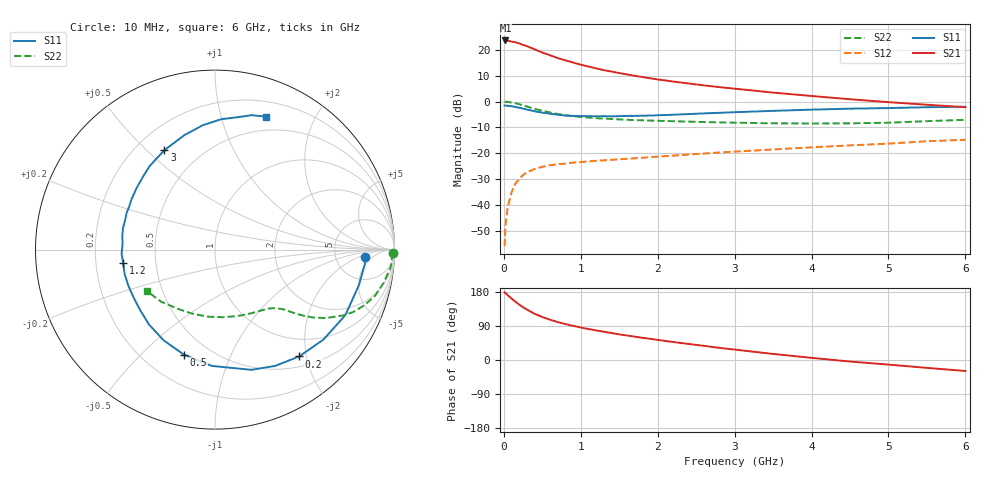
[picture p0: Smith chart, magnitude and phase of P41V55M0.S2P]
! SIEMENS Small Signal Semiconductors
! BFP182
! Si NPN RF Bipolar Junction Transistor in SOT143
! VCE = 1.5 V  IC = 5 mA
! Common Emitter S-Parameters:  March  1996
# GHz  S  MA  R  50
!  f  S11  S21  S12  S22
! GHz  MAG  ANG  MAG  ANG  MAG  ANG  MAG  ANG
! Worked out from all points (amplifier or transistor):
!   36 points, 10 MHz to 6 GHz, reference 50 ohm
!   highest |S21| = 23.6 dB at 20 MHz (marker M1)
!   |S21| within 3 dB of that: start of sweep to 364.8 MHz
!   unconditionally stable (mu >= 1): 1.537 GHz to 5.616 GHz
!   at 250 MHz: K = 0.22, MSG = 25.1 dB, |S12| = -28.4 dB
!   at 1.4 GHz: K = 0.95, MSG = 17.0 dB, |S12| = -22.5 dB
!   at 6 GHz: K = 0.96, MSG = 6.3 dB, |S12| = -14.8 dB
!   S11 on the Smith chart (normalised r, x): 10 MHz: 10, -3; 200 MHz: 0.67, -1.87; 500 MHz: 0.37, -0.68; 1.2 GHz: 0.32, -0.07; 3 GHz: 0.31, +0.57; 6 GHz: 0.35, +1.40
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0.01  0.8356 -2.8  14.93 178.4  0.0016 89.8  0.9898 -1.1
0.02  0.8386 -5.6  15.16 176.8  0.0039 89.9  0.9877 -2.2
0.05  0.8258 -13.9  15.03 170.9  0.0091 87.2  0.9838 -5.7
0.1  0.8129 -26.7  14.42 162.2  0.0176 74.6  0.9581 -11.1
0.15  0.785 -39.7  13.99 153.7  0.0257 68.8  0.9272 -16.2
0.2  0.7578 -51.8  13.29 146.1  0.0321 63.5  0.8874 -20.5
0.25  0.7299 -62.6  12.41 139.1  0.038 59.0  0.8464 -24.2
0.3  0.6996 -73.2  11.74 133.1  0.043 54.9  0.8023 -27.2
0.4  0.6484 -91.5  10.22 121.9  0.0496 48.0  0.7243 -31.8
0.5  0.6103 -106.5  8.845 113.4  0.0547 42.5  0.6623 -34.8
0.6  0.5809 -119.5  7.849 106.3  0.0587 39.6  0.6143 -36.8
0.7  0.5563 -131.4  6.928 100.2  0.0614 37.5  0.5759 -38.3
0.8  0.5365 -140.9  6.262 94.8  0.0632 35.5  0.5455 -39.5
1.1  0.5215 -164.9  4.748 81.7  0.0699 32.7  0.4896 -42.3
1.2  0.5174 -171.7  4.368 78.1  0.0716 32.0  0.4779 -43.4
1.7  0.5274 161.2  3.143 61.7  0.08 32.0  0.4371 -48.9
2.2  0.5557 141.7  2.436 47.5  0.0901 31.6  0.4165 -56.4
3  0.6219 116.9  1.773 27.5  0.1075 29.8  0.3899 -71.9
3.5  0.6605 104.9  1.489 16.0  0.1185 27.8  0.3793 -83.3
4.5  0.7275 87.2  1.108 -4.1  0.1419 22.9  0.3786 -109.3
5.5  0.7759 74.8  0.867 -20.8  0.1706 17.4  0.4172 -135.8
6  0.7939 69.0  0.777 -29.0  0.1824 13.1  0.4433 -148.3
